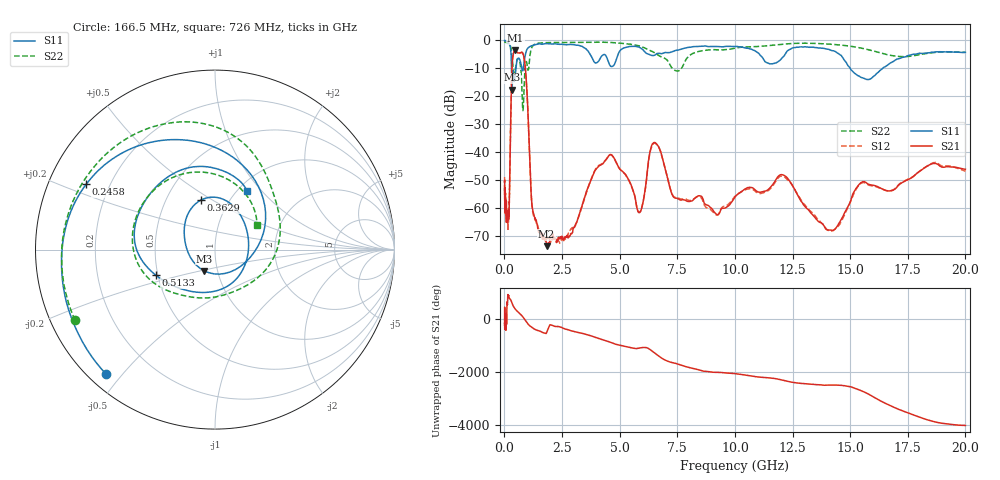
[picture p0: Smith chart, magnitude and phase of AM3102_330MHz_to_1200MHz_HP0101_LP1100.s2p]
! Date/Time: Tue, Sep 11, 2018 5:14 PM
! Network Analyzer: Agilent Technologies E8362B Rev: A.07.50.63
! Sweep from 0.010 to 20.000 GHz, 1601 Points, Sweep Type: LOG
! Power Supply: 4.949 V, 0.001 A
# Hz S DB R 50
!freq MagS11 AngS11 MagS21 AngS21 MagS12 AngS12 MagS22 AngS22
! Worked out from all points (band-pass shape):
!   1601 points, 10 MHz to 20 GHz, reference 50 ohm
!   highest |S21| = -3.58 dB at 475.7 MHz (marker M1); lowest = -73.5 dB at 1.833 GHz (marker M2)
!   |S21| within 3 dB of the highest: 353.4 MHz to 861.2 MHz (507.8 MHz wide, 83.6 % of centre)
!   lowest |S11| = -17.5 dB at 331.5 MHz (marker M3), VSWR 1.31, Z = 43.3 - j10.5 ohm
!   |S11| at or under -10 dB: 309.5 MHz to 500.5 MHz (190.9 MHz wide, 47.1 % of centre); 759 MHz to 821.5 MHz (62.55 MHz wide, 7.92 % of centre); 15 GHz to 16.4 GHz (1.4 GHz wide, 8.92 % of centre)
!   |S22| runs from -25.0 to -0.3 dB; largest |S21 - S12| = 0.012
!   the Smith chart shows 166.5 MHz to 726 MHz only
!   S11 on the Smith chart (normalised r, x): 166.5 MHz: 0.05, -0.45; 245.8 MHz: 0.11, +0.24; 362.9 MHz: 0.74, +0.44; 513.3 MHz: 0.49, -0.16; 726 MHz: 1.09, +0.83
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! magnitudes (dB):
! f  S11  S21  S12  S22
! 10 MHz  0.0  -50.5  -48.7  -0.3
! 35.55 MHz  0.0  -60.7  -61.7  -0.5
! 126.4 MHz  -0.4  -64.1  -62.3  -1.0
! 166.5 MHz  -0.7  -63.9  -65.5  -1.2
! 245.8 MHz  -1.9  -42.5  -42.7  -1.8
! 331.5 MHz  -17.5  -9.0  -9.1  -6.0
! 362.9 MHz  -10.9  -6.0  -6.1  -8.3
! 447.2 MHz  -13.7  -3.7  -3.7  -11.4
! 475.7 MHz  -12.1  -3.6  -3.6  -10.3
! 513.3 MHz  -8.9  -3.8  -3.9  -8.3
! 726 MHz  -8.6  -4.3  -4.3  -11.4
! 806 MHz  -10.6  -4.7  -4.8  -25.0
! 1.213 GHz  -1.9  -59.8  -60.3  -2.2
! 1.59 GHz  -1.3  -68.7  -69.3  -0.9
! 1.833 GHz  -1.1  -73.5  -71.1  -0.8
! 4.564 GHz  -8.7  -40.9  -40.8  -0.7
! 5.652 GHz  -2.1  -55.4  -55.4  -1.6
! 6.549 GHz  -5.1  -36.5  -36.7  -4.6
! 7.517 GHz  -3.5  -56.4  -56.2  -10.9
! 12.09 GHz  -5.9  -48.0  -48.5  -1.3
! 14.07 GHz  -3.2  -67.7  -67.9  -1.3
! 20 GHz  -4.3  -46.0  -46.7  -4.2
